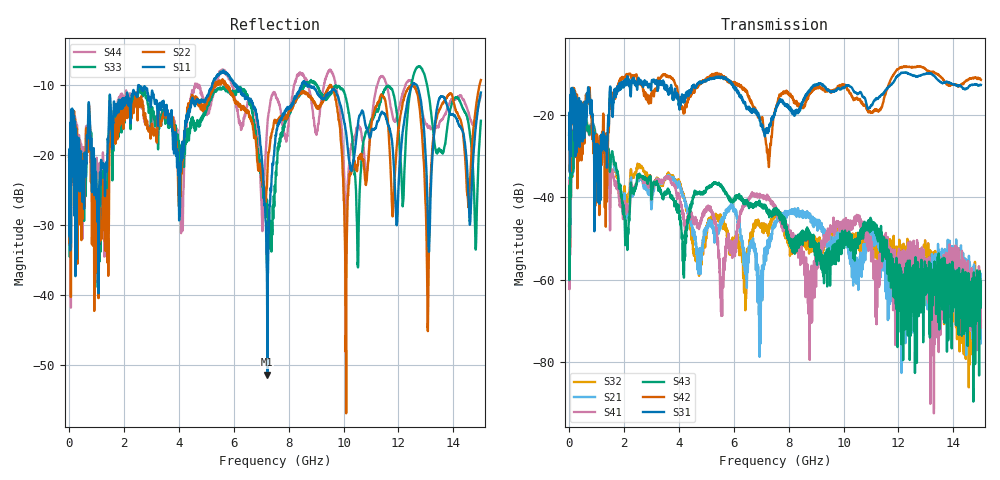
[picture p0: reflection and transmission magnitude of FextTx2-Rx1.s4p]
!  = SDD11
!  = SDD12
!  = SDC11
!  = SDC12
!  = SDD21
!  = SDD22
!  = SDC21
!  = SDC22
!  = SCD11
!  = SCD12
!  = SCC11
!  = SCC12
!  = SCD21
!  = SCD22
!  = SCC21
!  = SCC22
! FILE: N:\QM 2007\Prüfprotokolle\Highspeed\Konfektionierte Ltg\L45593-D106\D30\8216\0002\Fext\FextTx2-Rx1.s4p
# MHz S RI R 50.00
! FREQ  S11  S12  S13  S14
!  S21  S22  S23  S24
!  S31  S32  S33  S34
!  S41  S42  S43  S44
!  REAL  IMAG  REAL  IMAG  REAL  IMAG  REAL  IMAG
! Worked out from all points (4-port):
!   2999 points, 10 MHz to 15 GHz, reference 50 ohm
!   strongest paths, dB at 10 MHz, 3.755 GHz, 7.505 GHz, 11.26 GHz, 15 GHz:
!     S31: -24.9, -13.7, -19.5, -16.0, -12.8
!     S42: -24.6, -11.1, -19.1, -19.2, -11.6
!     S43: -46.9, -39.6, -42.8, -50.7, -60.6
!     S41: -46.5, -37.0, -42.4, -60.7, -71.5
!     S21: -50.6, -35.4, -46.7, -50.7, -65.9
!     S32: -40.7, -35.1, -43.6, -54.8, -69.9
!   lowest |S11| = -51.4 dB at 7.225 GHz (marker M1), VSWR 1.01, Z = 50.2 + j0.208 ohm
!   |S11| at or under -10 dB: start of sweep to 5.217 GHz; 6.105 GHz to 8.477 GHz (2.372 GHz wide, 32.5 % of centre); 8.672 GHz to 12.51 GHz (3.834 GHz wide, 36.2 % of centre)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
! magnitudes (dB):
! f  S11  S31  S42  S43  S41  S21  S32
! 10 MHz  -19.9  -24.9  -24.6  -46.9  -46.5  -50.6  -40.7
! 595 MHz  -20.5  -19.1  -21.2  -20.5  -20.8  -20.5  -20.2
! 2.11 GHz  -11.5  -12.7  -10.4  -48.1  -42.4  -43.3  -40.2
! 5.555 GHz  -8.2  -11.0  -10.8  -37.5  -68.3  -46.7  -45.0
! 7.225 GHz  -51.4  -23.4  -28.6  -43.7  -40.1  -53.8  -48.4
! 13.06 GHz  -28.5  -10.0  -9.4  -57.8  -65.0  -57.1  -52.6
! 15 GHz  -11.1  -12.8  -11.6  -60.6  -71.5  -65.9  -69.9
